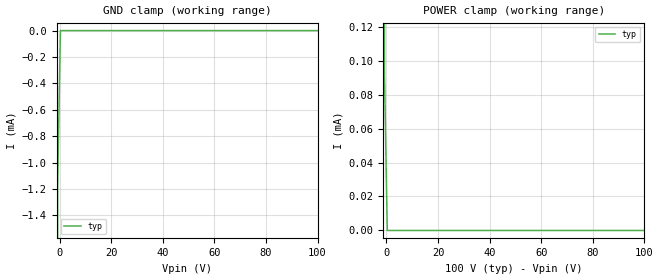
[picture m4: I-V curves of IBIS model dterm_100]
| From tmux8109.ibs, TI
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| dterm_100
[Model]   dterm_100
Model_type   Terminator
|   typ   min   max
C_comp   4.014581e-12   NA   NA
[Voltage Range]   100   NA   NA
[Temperature Range]   27   NA   NA
[Power Clamp Reference]   100   NA   NA
[GND Clamp Reference]   0   NA   NA
[GND Clamp]
|   Voltage   I(typ)   I(min)   I(max)
-5V       -2.258A    NA         NA
-1.818V   -237.5mA   NA         NA
-757.6mV  -1.165mA   NA         NA
303mV     -653.1pA   NA         NA
100V      3.307nA    NA         NA
[POWER Clamp]
|   Voltage   I(typ)   I(min)   I(max)
-5V       744mA      NA         NA
-1.818V   145.4mA    NA         NA
-758mV    90.5uA     NA         NA
303mV     3.301nA    NA         NA
100V      -690.1pA   NA         NA
